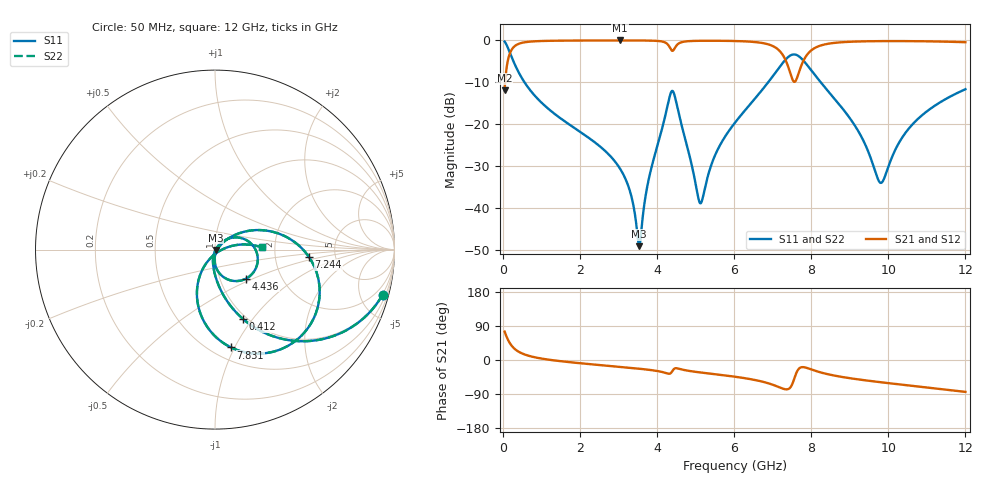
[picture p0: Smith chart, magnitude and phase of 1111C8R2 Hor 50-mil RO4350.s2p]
# GHz S MA R 50
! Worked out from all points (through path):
!   11951 points, 50 MHz to 12 GHz, reference 50 ohm
!   highest |S21| = -0.02 dB at 3.042 GHz (marker M1); lowest = -11.9 dB at 50 MHz (marker M2)
!   group delay of S21, straight-line fit = 20.7 ps
!   lowest |S11| = -49.0 dB at 3.542 GHz (marker M3), VSWR 1.01, Z = 50.3 - j0.162 ohm
!   |S11| at or under -10 dB: 566.6 MHz to 6.884 GHz (6.318 GHz wide, 170 % of centre); 8.249 GHz to end of sweep
!   |S22| runs from -49.0 to -0.3 dB; largest |S21 - S12| = 0
!   S11 on the Smith chart (normalised r, x): 50 MHz: 0.96, -7.45; 412 MHz: 0.96, -0.90; 4.436 GHz: 1.33, -0.46; 7.244 GHz: 3.17, -0.36; 7.831 GHz: 0.62, -0.97; 12 GHz: 1.71, +0.05
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0.05  0.9672 -15.0  0.254 74.9  0.254 74.9  0.9672 -15.0
0.187  0.713 -45.7  0.7008 44.2  0.7008 44.2  0.713 -45.7
0.412  0.418 -67.9  0.9078 22.0  0.9078 22.0  0.418 -67.9
2.042  0.07932 -97.9  0.9954 -8.9  0.9954 -8.9  0.07932 -97.9
3.042  0.02969 -104.2  0.9973 -18.2  0.9973 -18.2  0.02969 -104.2
3.318  0.01501 -100.7  0.9971 -20.8  0.9971 -20.8  0.01501 -100.7
3.542  0.003534 -27.1  0.9963 -23.0  0.9963 -23.0  0.003534 -27.1
3.76  0.01923 47.8  0.9941 -25.5  0.9941 -25.5  0.01923 47.8
4.034  0.0604 46.1  0.983 -29.5  0.983 -29.5  0.0604 46.1
4.436  0.2371 -42.8  0.7721 -24.3  0.7721 -24.3  0.2371 -42.8
5.125  0.01144 -29.3  0.9883 -32.8  0.9883 -32.8  0.01144 -29.3
5.517  0.04372 39.9  0.9893 -37.6  0.9893 -37.6  0.04372 39.9
6.025  0.1047 39.2  0.9821 -44.1  0.9821 -44.1  0.1047 39.2
7.244  0.5251 -4.5  0.6915 -74.8  0.6915 -74.8  0.5251 -4.5
7.561  0.6796 -45.6  0.3205 -49.6  0.3205 -49.6  0.6796 -45.6
7.831  0.5526 -80.7  0.609 -19.3  0.609 -19.3  0.5526 -80.7
8.017  0.4315 -95.9  0.7692 -25.4  0.7692 -25.4  0.4315 -95.9
9.177  0.08978 -122.7  0.9683 -50.6  0.9683 -50.6  0.08978 -122.7
9.769  0.02063 -68.5  0.9792 -58.2  0.9792 -58.2  0.02063 -68.5
10.009  0.03187 -7.0  0.9805 -61.1  0.9805 -61.1  0.03187 -7.0
10.704  0.1085 12.4  0.9778 -69.2  0.9778 -69.2  0.1085 12.4
12  0.2617 2.8  0.9505 -84.1  0.9505 -84.1  0.2617 2.8
